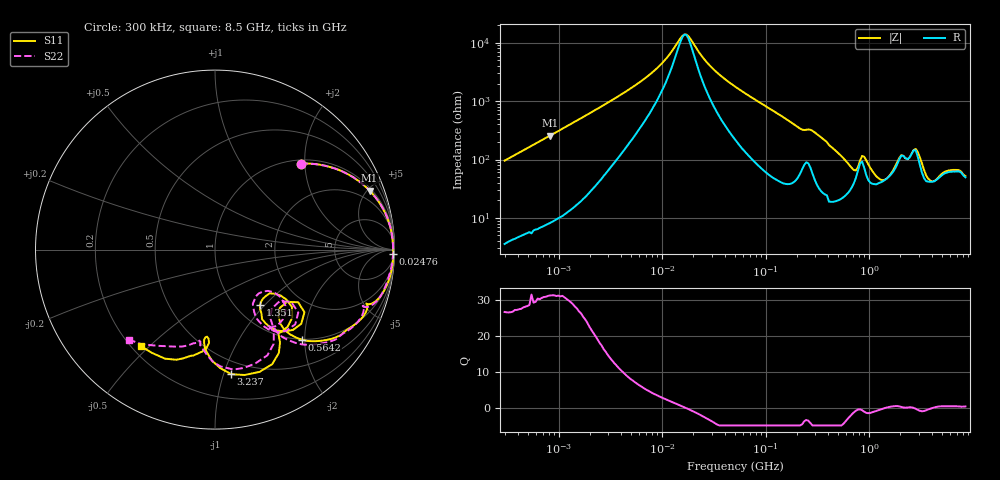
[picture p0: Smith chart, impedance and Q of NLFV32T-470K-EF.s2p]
! S-parameter Generated by TDK Corporation
! Copyright(C) 2015 TDK Corporation.
! All Rights Reserved.
! TDK P/N: NLFV32T-470K-EF (Inductors)
! Property: L=47uH at 2.52MHz
! Size(LxWxT): 3.2x2.5x2.2mm, 0.126x0.098x0.087inches
! Model Type: s2p (Touchstone File Format Version 1.0)
! Frequency: DC=Yes Start=0.3MHz Stop=8500MHz 225points Log-sweep
! Note:
! Model Generated on Jun. 23, 2015
! Hash(MD5):
! Port Assignments:
!  1 ---@@@--- 2
! Applicable Conditions:
!  Temperature = 25 degC
!  DC Bias Current = 0 A
!  Small Signal Operation
! Terms and conditions regarding TDK Simulation Models
! (1)This simulation model is being provided solely for informational purposes. Please refer to the specifications of the products in terms of detailed characteristics of such products.
! (2)In no event shall TDK Corporation of any of its subsidiaries be liable for any loss or damage arising, directly or indirectly,
!  From any information contained in this simulation model, including, but not limited to loss or damages arising from any inaccuracies, omissions or errors in connection with such information.
! (3)Any and all copyrights on this simulation model are owned by TDK Corporation.
!  Duplication or redistribution of this simulation model without prior written permission from TDK Corporation is prohibited.
! (4)This simulation model is subject to any modification or change without any prior notice.
! (5)Neither TDK Corporation nor any of its subsidiaries shall make any warranty, express or implied,
!  Including but not limited to the correctness, implied warranties of merchantability and fitness for a particular purpose with respect to this simulation models.
! (6)The use of this simulation model shall be deemed to have consented to the terms and conditions hereof.
# MHz S MA R 50
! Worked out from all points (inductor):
!   224 points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, 300 kHz to 8.5 GHz, reference 50 ohm
!   read as one part in series: L = 50.4 uH near 314.1 kHz
!   highest Q = 31.3 at 824.8 kHz (marker M1), where L = 49.5 uH
!   self-resonance near 16.37 MHz
!   S11 on the Smith chart (normalised r, x): 300 kHz: 1.08, +1.91; 24.76 MHz: 20, -75; 564.2 MHz: 0.99, -1.93; 1.351 GHz: 1.28, -0.94; 3.237 GHz: 0.39, -1.06; 8.5 GHz: 0.24, -0.47
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0.3  0.6775 45.0  0.7089 -42.8  0.7147 -43.0  0.6759 45.0
0.8248242  0.9219 20.9  0.3594 -67.3  0.3608 -67.6  0.9221 20.9
1.72111  0.976 10.4  0.1828 -77.4  0.1834 -77.7  0.9769 10.4
9.430415  0.9922 1.2  0.02458 -70.9  0.0246 -71.2  0.9921 1.0
16.37255  0.993 -0.3  0.007161 -4.7  0.007159 -5.1  0.9927 -0.5
24.76313  0.9935 -1.4  0.0179 66.2  0.01791 66.0  0.9926 -1.7
51.67171  0.9928 -4.2  0.05724 78.7  0.05724 78.4  0.9896 -4.6
205.2186  0.9329 -18.4  0.2571 63.1  0.2573 62.8  0.9246 -19.7
283.1228  0.9101 -21.5  0.2863 57.4  0.2865 57.1  0.8971 -22.8
564.2308  0.6968 -46.1  0.5934 31.2  0.5933 30.9  0.6857 -49.2
778.4218  0.4951 -36.0  0.5742 1.2  0.574 0.9  0.4609 -38.6
853.3868  0.6084 -35.0  0.4671 6.3  0.4678 5.9  0.5816 -37.1
979.5854  0.5956 -49.9  0.5799 11.8  0.5792 11.3  0.5726 -53.1
1351.452  0.3994 -51.1  0.6629 -12.2  0.6634 -12.5  0.3685 -55.1
1551.304  0.3839 -42.1  0.6344 -23.3  0.635 -24.0  0.3452 -44.9
2044.041  0.5738 -41.4  0.423 -36.4  0.4233 -36.6  0.5412 -44.0
2693.286  0.6764 -58.2  0.3434 -37.3  0.3435 -38.1  0.6182 -58.0
3237.012  0.6997 -82.6  0.4355 -20.3  0.436 -21.0  0.6762 -81.3
3715.7  0.587 -93.7  0.5272 -34.1  0.5283 -34.5  0.5919 -94.1
4675.929  0.4871 -95.2  0.5136 -58.5  0.515 -59.2  0.5167 -99.5
7072.242  0.6314 -106.3  0.3469 -86.1  0.3484 -86.8  0.6196 -120.0
8500  0.6779 -127.7  0.2915 -96.8  0.291 -96.1  0.6944 -133.4
